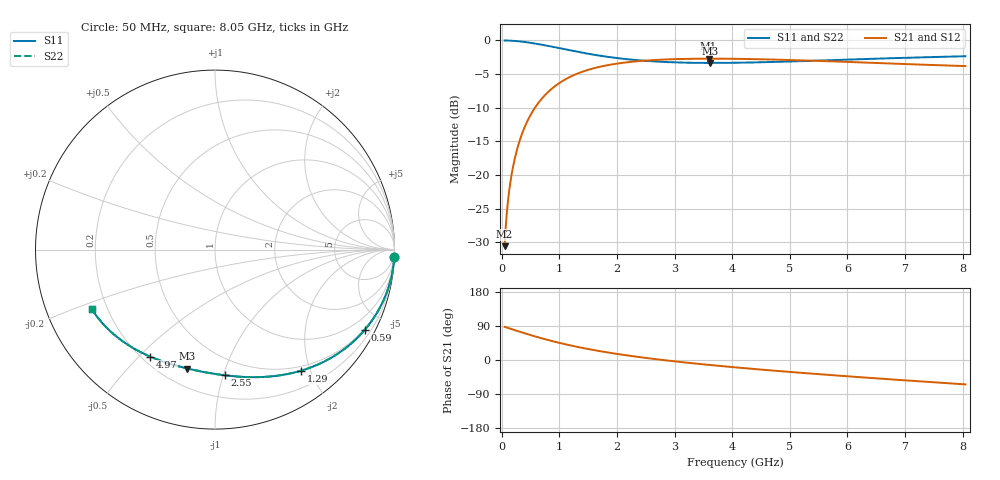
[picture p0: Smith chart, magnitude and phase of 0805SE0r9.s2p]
! AVX Thin Film Operation		Date: August 2001
! Description: Accu-P® Series, Thin Film, SMD, RF Capacitor
! Part Number: 08051J0R9ABT
! 50 MHz  -  8.05 GHz
! Serial Measurements
# mhz S db R 50
!	S11		S21		S12		S22
!	dB	Phase	dB	Phase	dB	Phase	dB	Phase
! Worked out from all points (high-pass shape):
!   401 points, 50 MHz to 8.05 GHz, reference 50 ohm
!   highest |S21| = -2.71 dB at 3.59 GHz (marker M1); lowest = -30.6 dB at 50 MHz (marker M2)
!   |S21| within 3 dB of the highest: 1.121 GHz to end of sweep
!   lowest |S11| = -3.3 dB at 3.61 GHz (marker M3), VSWR 5.26, Z = 15.2 - j37.4 ohm
!   |S11| at or under -10 dB: nowhere
!   |S22| runs from -3.3 to 0.0 dB; largest |S21 - S12| = 0
!   S11 on the Smith chart (normalised r, x): 50 MHz: 0, -46; 590 MHz: 0.46, -3.93; 1.29 GHz: 0.43, -1.86; 2.55 GHz: 0.37, -1.01; 4.97 GHz: 0.23, -0.54; 8.05 GHz: 0.14, -0.22
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50  -0.00 -2.5  -30.57 87.5  -30.57 87.5  -0.00 -2.5
70  -0.01 -3.5  -27.66 86.5  -27.66 86.5  -0.01 -3.5
110  -0.02 -5.5  -23.75 84.5  -23.75 84.5  -0.02 -5.5
150  -0.03 -7.5  -21.08 82.5  -21.08 82.5  -0.03 -7.5
190  -0.05 -9.4  -19.05 80.6  -19.05 80.6  -0.05 -9.4
250  -0.09 -12.4  -16.73 77.6  -16.73 77.6  -0.09 -12.4
390  -0.22 -19.1  -13.05 70.9  -13.05 70.9  -0.22 -19.1
590  -0.48 -28.2  -9.84 61.8  -9.84 61.8  -0.48 -28.2
730  -0.69 -34.2  -8.32 55.8  -8.32 55.8  -0.69 -34.2
910  -0.99 -41.4  -6.89 48.6  -6.89 48.6  -0.99 -41.4
1290  -1.65 -54.7  -5.01 35.3  -5.01 35.3  -1.65 -54.7
1390  -1.81 -57.8  -4.68 32.2  -4.68 32.2  -1.81 -57.8
1930  -2.54 -72.3  -3.54 17.7  -3.54 17.7  -2.54 -72.3
2550  -3.06 -85.4  -2.96 4.5  -2.96 4.5  -3.06 -85.4
2730  -3.16 -88.8  -2.87 1.2  -2.87 1.2  -3.16 -88.8
3590  -3.35 -102.8  -2.71 -12.8  -2.71 -12.8  -3.35 -102.8
3610  -3.35 -103.1  -2.71 -13.1  -2.71 -13.1  -3.35 -103.1
4050  -3.32 -109.3  -2.73 -19.3  -2.73 -19.3  -3.32 -109.3
4970  -3.14 -121.1  -2.90 -31.1  -2.90 -31.1  -3.14 -121.1
5390  -3.02 -126.0  -3.01 -36.1  -3.01 -36.1  -3.02 -126.0
6730  -2.65 -140.7  -3.42 -50.8  -3.42 -50.8  -2.65 -140.7
8050  -2.35 -154.3  -3.81 -64.4  -3.81 -64.4  -2.35 -154.3
